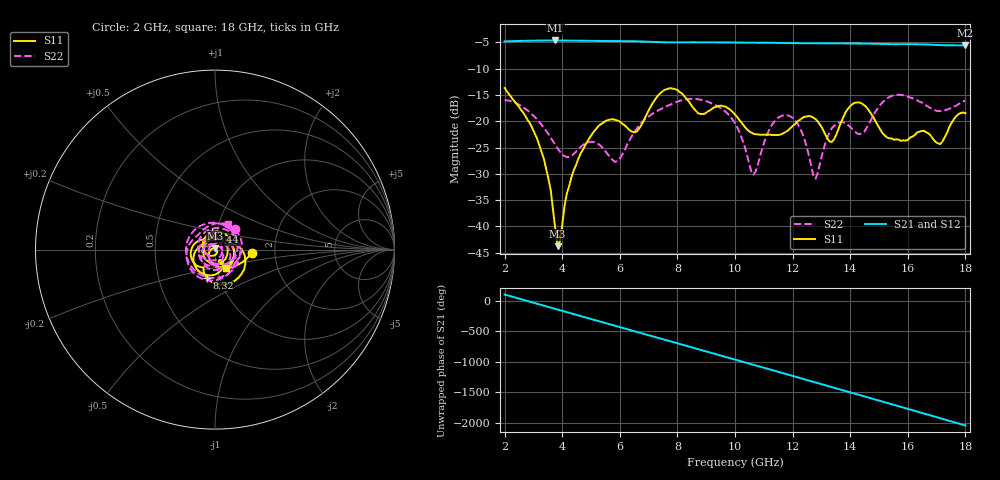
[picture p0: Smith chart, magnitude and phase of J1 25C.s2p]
!Agilent Technologies,E8363B,SG43030131,A.07.50.48
!Agilent E8363B: A.07.50.48
!Date: Wednesday, December 17, 2025 22:17:12
!Correction: S11(Full 2 Port(1,2))
!S21(Full 2 Port(1,2))
!S12(Full 2 Port(1,2))
!S22(Full 2 Port(1,2))
!S2P File: Measurements: S11, S21, S12, S22:
# Hz S  dB  R 50
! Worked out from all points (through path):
!   201 points, 2 GHz to 18 GHz, reference 50 ohm
!   highest |S21| = -4.63 dB at 3.76 GHz (marker M1); lowest = -5.6 dB at 18 GHz (marker M2)
!   group delay of S21, straight-line fit = 371 ps
!   lowest |S11| = -43.8 dB at 3.84 GHz (marker M3), VSWR 1.01, Z = 50.1 + j0.642 ohm
!   |S11| at or under -10 dB: start of sweep to end of sweep
!   |S22| runs from -30.9 to -14.9 dB; largest |S21 - S12| = 0.0013
!   S11 on the Smith chart (normalised r, x): 2 GHz: 1.52, -0.06; 5.44 GHz: 0.95, +0.18; 8.32 GHz: 0.87, -0.28; 18 GHz: 1.11, -0.23
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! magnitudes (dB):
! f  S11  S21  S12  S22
! 2 GHz  -13.7  -4.8  -4.8  -16.0
! 3.12 GHz  -23.2  -4.7  -4.7  -19.6
! 3.6 GHz  -33.1  -4.6  -4.6  -23.2
! 3.76 GHz  -40.5  -4.6  -4.6  -24.5
! 3.84 GHz  -43.8  -4.6  -4.6  -25.2
! 4.16 GHz  -33.8  -4.7  -4.6  -26.8
! 4.72 GHz  -25.4  -4.7  -4.7  -24.5
! 5.44 GHz  -20.2  -4.7  -4.7  -25.3
! 5.92 GHz  -19.9  -4.8  -4.7  -27.6
! 6.56 GHz  -22.1  -4.8  -4.8  -21.6
! 7.36 GHz  -14.9  -5.0  -5.0  -17.8
! 8.32 GHz  -15.8  -5.0  -5.0  -15.8
! 10 GHz  -18.7  -5.0  -5.0  -20.4
! 10.64 GHz  -22.4  -5.1  -5.1  -30.2
! 11.28 GHz  -22.6  -5.1  -5.1  -20.7
! 12 GHz  -20.9  -5.1  -5.1  -19.4
! 12.72 GHz  -19.3  -5.2  -5.2  -30.3
! 13.44 GHz  -23.4  -5.2  -5.2  -20.9
! 14.24 GHz  -16.4  -5.2  -5.2  -22.3
! 15.36 GHz  -23.3  -5.3  -5.3  -15.4
! 17.12 GHz  -24.4  -5.5  -5.5  -18.1
! 18 GHz  -18.5  -5.6  -5.6  -16.0
